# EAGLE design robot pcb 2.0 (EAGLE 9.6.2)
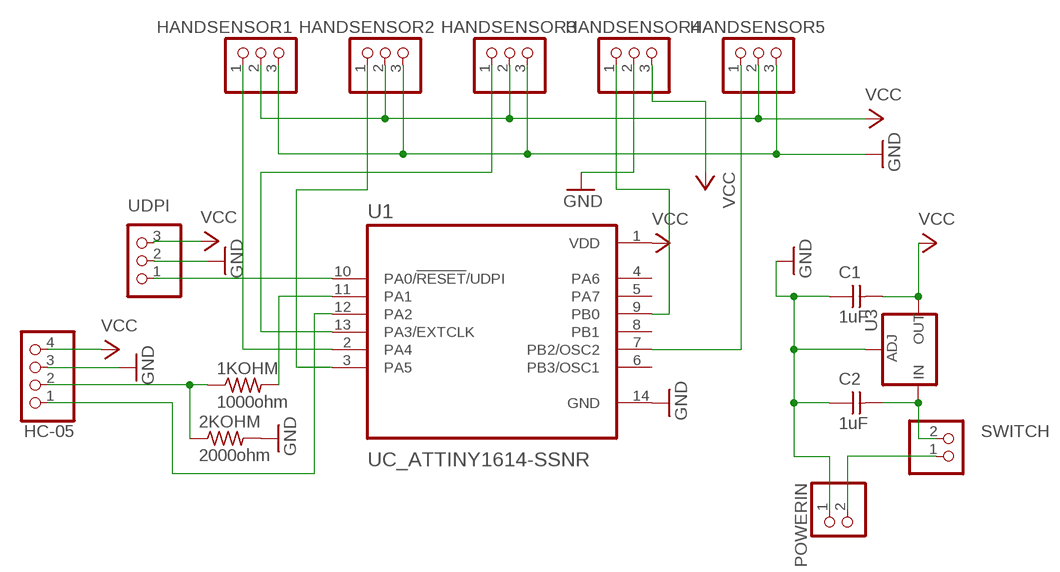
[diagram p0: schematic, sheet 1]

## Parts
1KOHM  1000ohm  R1206FAB  [R1206FAB]
2KOHM  2000ohm  R1206FAB  [R1206FAB]
C1  1uF  CAP_UNPOLARIZEDFAB  [C1206FAB]
C2  1uF  CAP_UNPOLARIZEDFAB  [C1206FAB]
HANDSENSOR1  PINHD-1X3  [1X03]
HANDSENSOR2  PINHD-1X3  [1X03]
HANDSENSOR3  PINHD-1X3  [1X03]
HANDSENSOR4  PINHD-1X3  [1X03]
HANDSENSOR5  PINHD-1X3  [1X03]
HC-05  PINHD-1X4  [1X04]
POWERIN  PINHD-1X2  [1X02]
SWITCH  PINHD-1X2  [1X02]
U1  UC_ATTINY1614-SSNR  [SOIC127P600X175-14N]
U3  V_REG_LM1117SOT223  [SOT223]
UDPI  PINHD-1X3  [1X03]

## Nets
GND: 2KOHM.2 C1.1 C2.1 HANDSENSOR1.3 HANDSENSOR2.3 HANDSENSOR3.3 HANDSENSOR4.2 HANDSENSOR5.3 HC-05.3 POWERIN.1 U1.14(GND) U3.1(ADJ) UDPI.2
N$1: HANDSENSOR1.1 U1.2(PA4)
N$2: HANDSENSOR2.1 U1.3(PA5)
N$3: U1.10(PA0/!RESET!/UDPI) UDPI.1
N$4: HC-05.1 U1.12(PA2)
N$5: 1KOHM.1 2KOHM.1 HC-05.2
N$6: C2.2 SWITCH.2 U3.3(IN)
N$7: POWERIN.2 SWITCH.1
N$10: 1KOHM.2 U1.11(PA1)
N$12: HANDSENSOR3.1 U1.13(PA3/EXTCLK)
N$13: HANDSENSOR4.1 U1.9(PB0)
N$14: HANDSENSOR5.1 U1.7(PB2/OSC2)
VCC: C1.2 HANDSENSOR1.2 HANDSENSOR2.2 HANDSENSOR3.2 HANDSENSOR4.3 HANDSENSOR5.2 HC-05.4 U1.1(VDD) U3.2(OUT) U3.4(OUT) UDPI.3
Unconnected: U1.4(PA6) U1.5(PA7) U1.6(PB3/OSC1) U1.8(PB1)

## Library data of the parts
1KOHM 2KOHM = fab:R: Resistor (US Symbol)
C1 C2 = fab:CAP_UNPOLARIZED
HANDSENSOR1-HANDSENSOR5 UDPI = pinhead:PINHD-1X3: PIN HEADER
HC-05 = pinhead:PINHD-1X4: PIN HEADER
POWERIN SWITCH = pinhead:PINHD-1X2: PIN HEADER
U1 = fab:UC_ATTINY1614-SSNR: 20MHz, SOIC, 85C, Green, 14 SOIC .150in T/R Check prices; AVAILABILITY: In Stock; DESCRIPTION: AVR tinyAVR™ 1, Functional Safety (FuSa) Microcontroller IC 8-Bit 20MHz 16KB (16K x 8) FLASH 14-SOIC; MF: Microchip Technology; MP: ATTINY1614-SSNR; PACKAGE: None; PRICE: None; PURCHASE-URL: https://pricing.snapeda.com/search/part/ATTINY1614-SSNR/?ref=eda
U3 = SparkFun-IC-Power:V_REG_LM1117: Voltage Regulator LM1117 Standard adjustable voltage regulator but in SMD form. Spark Fun Electronics SKU : COM-00595; PROD_ID: VREG-08170

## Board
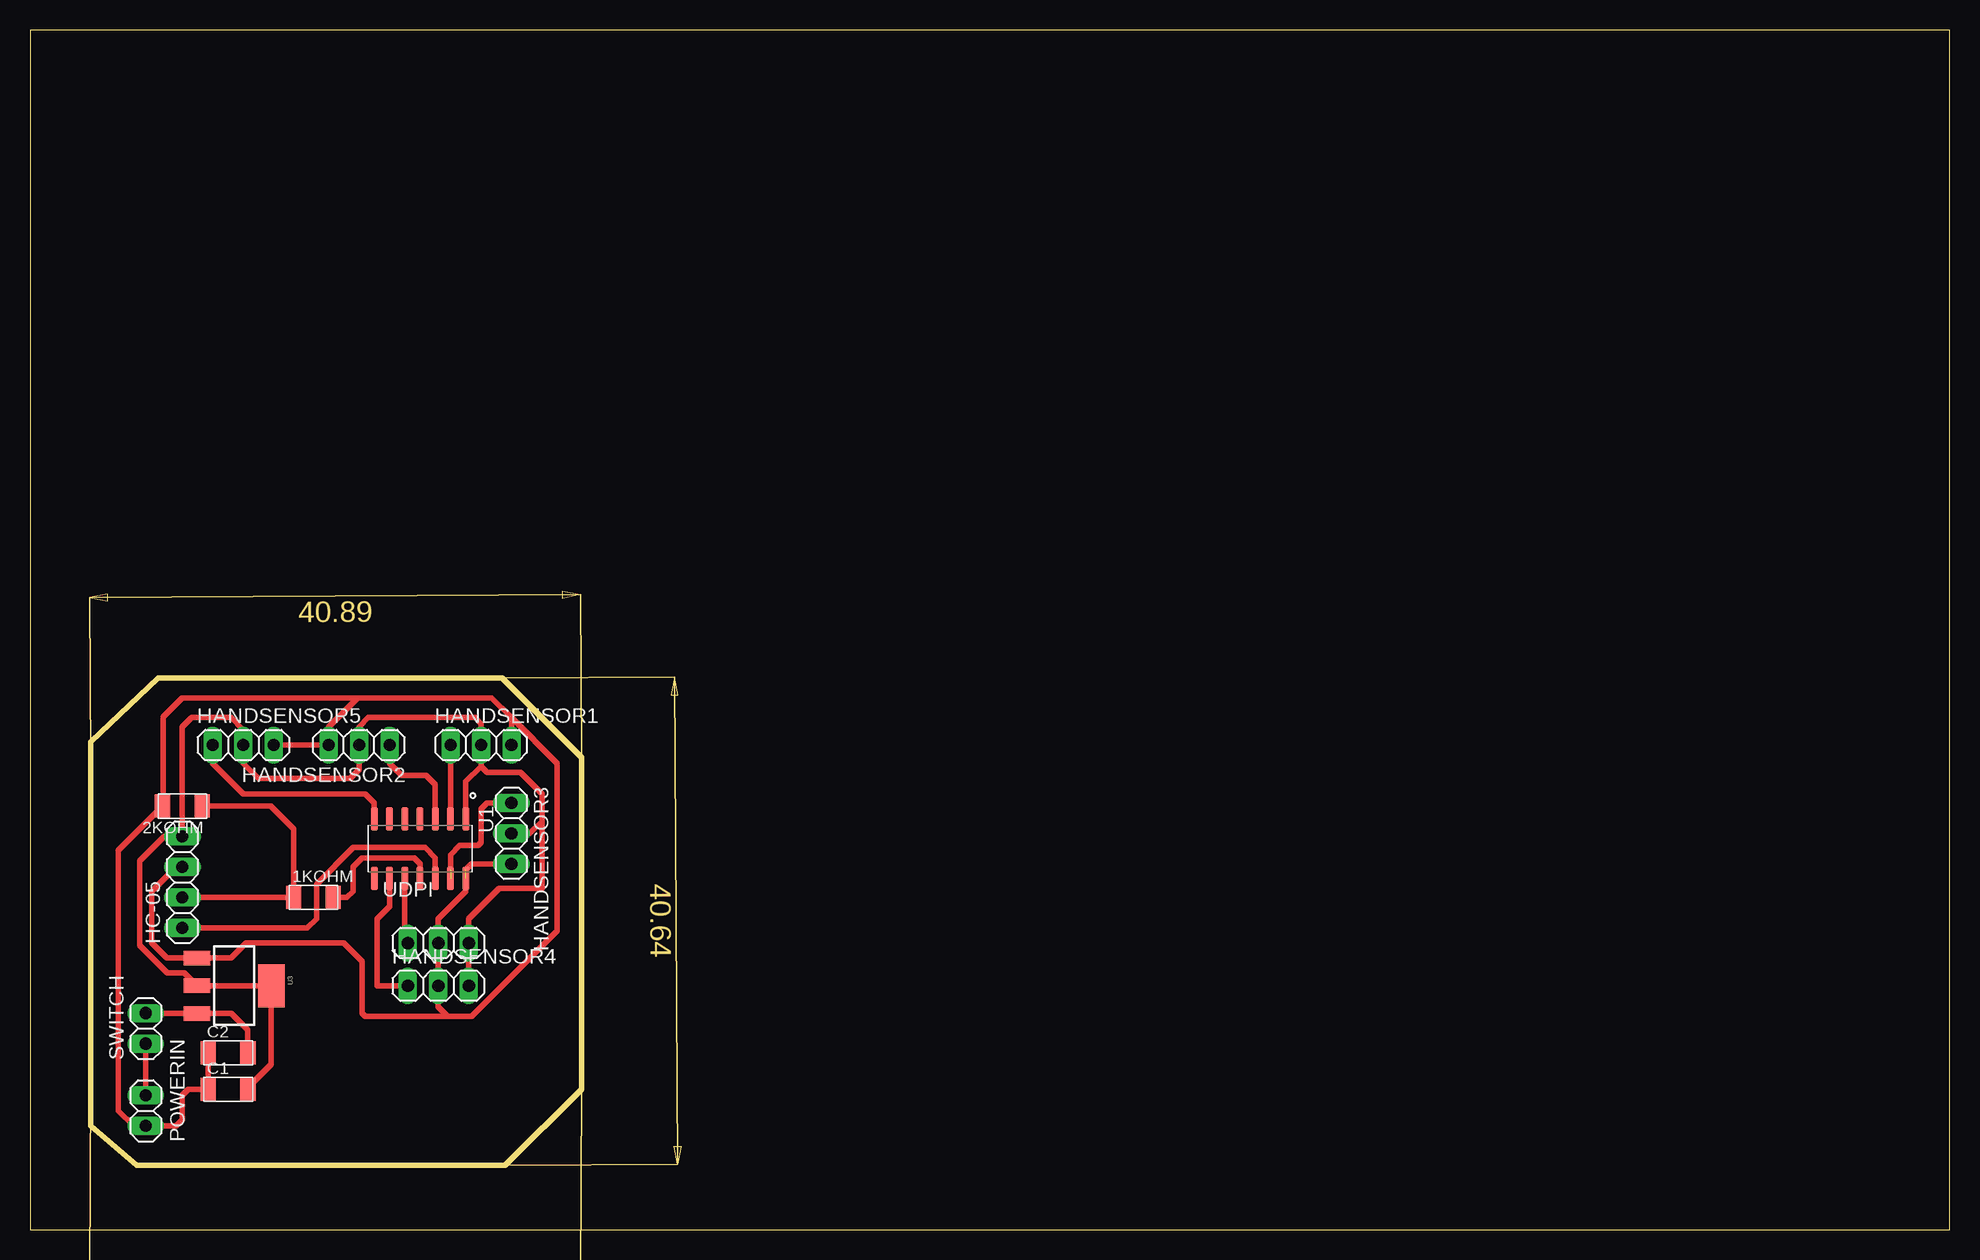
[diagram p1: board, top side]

Size 160 x 100 mm. Coordinates in mm from the lower left corner, seen from the top.
Outline: 0,0 160,0 160,100 0,100 0,0
Copper layers (1*16): Top 0.035mm / dielectric 1.5mm / Bottom 0.035mm
Design rules "default *": minimum track width 18mil, minimum drill 0.35mm, track to track 16mil, track to pad 16mil, pad to pad 16mil, via to via 12mil, smd to smd 10mil, copper to edge 40mil, drill to drill 6mil, minimum pad ring 10mil, minimum via ring 8mil, stop-mask expansion 4mil, vias tented up to drill 0mil, thermal gap 10mil
Milling: area 53.7,5.4 to 54.3,6.9; area 53.4,44.6 to 54,46.1; area 51.7,22.3 to 53.5,29.2; area 44.4,52.6 to 45.9,53.2; area 5,52.4 to 6.5,53; area 22,50.6 to 28.9,52.4; area 44.4,-4.2 to 45.9,-3.6; area 5,-4 to 6.5,-3.4; area 21.9,-6 to 28.9,-4.2; 17 lines

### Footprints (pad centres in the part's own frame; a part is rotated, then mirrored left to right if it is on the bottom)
R1206FAB = smd 1.27 x 1.905: 1 -1.651,0; 2 1.651,0
C1206FAB = smd 1.27 x 1.905: 1 -1.651,0; 2 1.651,0
1X03 = drill 1.016 long: 1 -2.54,0; 2 0,0; 3 2.54,0
1X04 = drill 1.016 long: 1 -3.81,0; 2 -1.27,0; 3 1.27,0; 4 3.81,0
1X02 = drill 1.016 long: 1 -1.27,0; 2 1.27,0
SOIC127P600X175-14N = smd 1.95 x 0.59: 1 -2.48,3.81; 2 -2.48,2.54; 3 -2.48,1.27; 4 -2.48,0; 5 -2.48,-1.27; 6 -2.48,-2.54; 7 -2.48,-3.81; 8 2.48,-3.81; 9 2.48,-2.54; 10 2.48,-1.27; 11 2.48,0; 12 2.48,1.27; 13 2.48,2.54; 14 2.48,3.81
SOT223 = smd 1.219 x 2.235: 1 -2.311,-3.099; 2 0,-3.099; 3 2.311,-3.099 | smd 3.6 x 2.2: 4 0,3.099

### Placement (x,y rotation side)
1KOHM  23.62,27.69 0 top
2KOHM  12.7,35.31 180 top
C1  16.51,11.68 0 top
C2  16.51,14.73 0 top
HANDSENSOR1  37.59,40.39 0 top
HANDSENSOR2  27.43,40.39 180 top
HANDSENSOR3  40.13,33.02 270 top
HANDSENSOR4  34.04,20.32 0 top
HANDSENSOR5  17.78,40.39 0 top
HC-05  12.7,28.96 90 top
POWERIN  9.65,9.91 90 top
SWITCH  9.65,16.76 90 top
U1  32.51,31.75 270 top
U3  17.02,20.32 270 top
UDPI  34.04,23.88 0 top

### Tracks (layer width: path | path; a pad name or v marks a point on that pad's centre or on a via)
GND  (1 unrouted)
  Top 0.457: HANDSENSOR1.3 40.13,42.67 | 36.32,28.45 U1.14 36.32,28.19 34.04,25.91 UDPI.2 HANDSENSOR4.2 34.04,18.54 34.8,17.78 | 40.13,42.67 38.48,44.32 27.3,44.32 | 27.3,44.32 24.89,41.91 HANDSENSOR2.3 HANDSENSOR5.3 | 27.3,44.32 12.7,44.32 11.11,42.74 11.11,35.37 2KOHM.2 7.37,31.62 7.37,9.91 8.64,8.64 POWERIN.1 12.19,8.64 12.7,9.14 12.7,11.18 13.21,11.68 C1.1 C2.1 | 41.4,30.48 HANDSENSOR3.3 36.83,30.48 36.32,29.97 | HC-05.3 12.19,30.23 10.16,28.19 10.16,23.88 11.4,22.63 U3.1 16.79,22.63 18.03,23.88 26.16,23.88 27.69,22.35 27.69,18.03 27.94,17.78 34.8,17.78 | 40.13,42.67 43.94,38.86 43.94,24.89 36.83,17.78 34.8,17.78
N$1
  Top 0.457: HANDSENSOR1.1 U1.2
N$2
  Top 0.457: U1.3 33.78,37.08 33.02,37.85 30.99,37.85 29.97,38.86 HANDSENSOR2.1
N$3
  Top 0.457: UDPI.1 31.24,24.13 U1.10
N$4
  Top 0.457: U1.12 33.78,30.99 32.92,31.85 26.95,31.85 23.88,28.77 23.88,25.91 23.11,25.15 HC-05.1
N$5
  Top 0.457: 14.35,35.28 2KOHM.1 20.07,35.31 21.97,33.4 1KOHM.1 HC-05.2
N$6
  Top 0.457: SWITCH.2 13.69,18.03 13.82,17.91 U3.3 16.74,18.01 16.76,18.03 18.16,16.64 C2.2
N$7
  Top 0.457: POWERIN.2 SWITCH.1
N$10
  Top 0.457: U1.11 32.51,30.48 32,30.99 27.69,30.99 26.92,30.23 26.92,28.19 26.42,27.69 1KOHM.2
N$12  (1 unrouted)
  Top 0.457: HANDSENSOR3.1 38.1,35.56 37.59,35.05 37.59,32.26 37.34,32 35.81,32 35.05,31.24 35.05,29.97
N$13
  Top 0.457: HANDSENSOR4.1 28.96,20.32 28.96,25.91 29.97,26.92 U1.9
N$14
  Top 0.457: U1.7 28.7,35.56 27.94,36.32 17.78,36.32 15.24,38.86 HANDSENSOR5.1
VCC
  Top 0.457: 37.59,39.37 HANDSENSOR1.2 | HANDSENSOR1.2 37.59,42.16 37.08,42.67 28.19,42.67 27.43,41.91 HANDSENSOR2.2 27.43,38.35 26.67,37.59 19.05,37.59 17.78,38.86 HANDSENSOR5.2 17.78,41.66 16.76,42.67 13.46,42.67 12.7,41.91 HC-05.4 11.18,32.77 9.14,30.73 9.14,23.67 11.43,21.39 12.85,21.39 U3.2 U3.4 20.12,13.77 18.16,11.81 C1.2 | HANDSENSOR1.2 37.59,38.61 | U1.1 36.32,37.34 37.59,38.61 | 17.78,11.3 C1.2 | 18.03,11.56 C1.2 | 37.59,38.61 38.1,38.1 40.89,38.1 42.67,36.32 42.67,34.04 | HANDSENSOR3.2 41.66,33.02 42.67,34.04 | 42.67,34.04 42.67,28.45 39.12,28.45 36.58,25.91 UDPI.3 HANDSENSOR4.3

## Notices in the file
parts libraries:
SparkFun-IC-Power: Licensing: Creative Commons ShareAlike 4.0 International - https://creativecommons.org/licenses/by-sa/4.0
